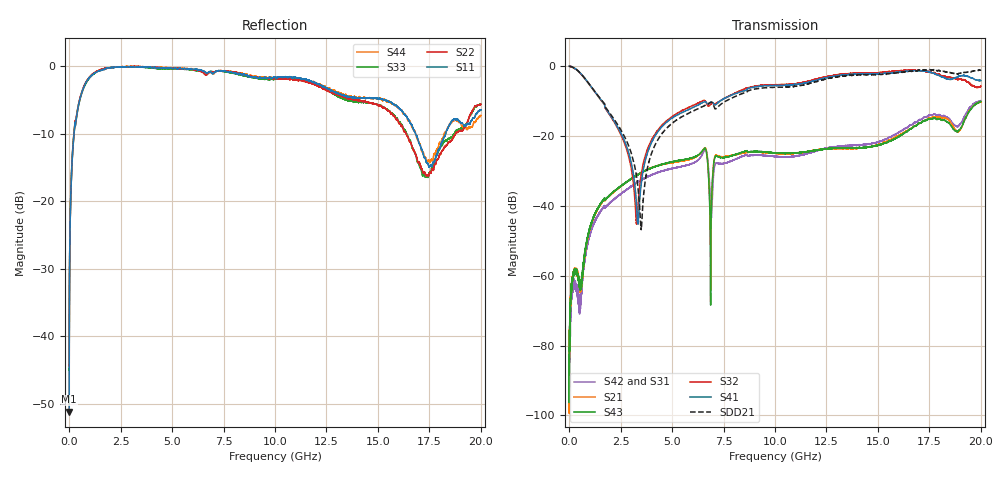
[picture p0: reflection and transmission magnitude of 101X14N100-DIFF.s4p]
!{101X14N100}
!Johanson Technology Inc.
!www.johansontechnology.com
!Test Board Conditions:
!Substrate Type  RO4350B
!Substrate Thickness  10 mil
!Substrate Dk  3.66
!TL Type: GCPW
!TL Trace Width  20 mil
!TL Gap  15 mil
!PART MODE DIFFERENTIAL
!DUT TOPOLOGY	DIFFERENTIAL 4-PORT
!Mounting Pad LxW  20x35 mil
# MHz S  dB  R 50
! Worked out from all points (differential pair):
!   20001 points, 300 kHz to 20 GHz, reference 50 ohm
!   strongest paths, dB at 300 kHz, 5 GHz, 10 GHz, 15 GHz, 20 GHz:
!     S41: 0.0, -14.9, -5.5, -2.2, -4.1
!     S32: 0.0, -14.5, -5.3, -1.9, -5.7
!     S43: -87.1, -27.4, -24.8, -22.7, -10.1
!     S21: -85.9, -27.6, -24.9, -22.6, -10.3
!     S42: -80.8, -29.3, -25.8, -21.8, -9.9
!     S31: -74.6, -29.4, -25.7, -21.8, -10.1
!   taken as a pair (ports 1,2 in; 4,3 out), SDD21 dB: 0.0, -16.4, -6.0, -2.4, -1.1
!   lowest |S11| = -51.1 dB at 1.3 MHz (marker M1), VSWR 1.01, Z = 50.1 - j0.254 ohm
!   |S11| at or under -10 dB: start of sweep to 237.8 MHz; 16.83 GHz to 18.29 GHz (1.46 GHz wide, 8.32 % of centre); 18.28786 GHz to 18.28805 GHz (187.9 kHz wide, 0.00103 % of centre)
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0.3  -51.00 -16.2  -85.28 164.2  -79.63 16.6  -0.00 -0.2
     -85.92 -132.7  -44.18 2.4  -0.01 -0.2  -87.12 -155.3
     -74.56 -13.4  -0.03 -0.3  -44.80 -2.9  -80.59 -88.7
     0.00 -0.1  -80.80 68.5  -87.15 159.6  -51.02 -17.7
1.3  -51.14 -66.0  -87.85 125.6  -86.01 -99.6  -0.01 -0.2
     -99.38 -95.9  -44.41 -22.0  -0.06 -0.0  -84.72 -100.0
     -87.78 115.0  -0.05 -0.1  -45.09 -22.9  -81.50 -7.1
     -0.01 -0.2  -87.43 -83.0  -84.25 -17.6  -51.38 -65.2
553.292  -4.49 -131.2  -64.54 81.3  -67.35 -105.6  -1.99 -41.7
         -64.19 74.3  -4.41 -133.0  -2.12 -42.6  -67.09 -102.9
         -66.08 -93.6  -2.11 -42.7  -4.60 -133.0  -62.52 85.2
         -2.00 -41.8  -66.23 -91.1  -62.55 89.7  -4.46 -133.3
3343.25  -0.10 171.4  -30.99 77.8  -33.10 76.9  -44.96 -10.0
         -31.01 77.7  -0.05 168.5  -40.21 42.8  -33.20 76.8
         -33.17 77.3  -40.23 42.9  -0.08 167.5  -31.09 76.7
         -45.09 -10.6  -33.18 76.9  -31.10 76.5  -0.09 169.3
6516.202  -0.72 134.6  -23.86 10.7  -24.71 1.5  -10.32 37.1
          -23.90 10.7  -0.93 131.3  -9.87 32.4  -24.75 -0.1
          -24.71 1.6  -9.85 32.8  -0.92 127.8  -23.89 7.2
          -10.33 37.1  -24.75 0.4  -23.92 7.2  -0.79 129.6
6875.197  -0.84 136.8  -63.98 173.3  -39.23 -123.6  -10.30 32.6
          -63.07 179.9  -0.83 129.2  -10.94 29.6  -39.67 -125.2
          -39.16 -122.4  -10.96 29.7  -0.77 126.3  -62.44 65.4
          -10.28 32.9  -39.79 -124.3  -61.21 72.2  -0.91 126.5
20000  -6.44 72.7  -10.26 104.5  -10.13 105.7  -4.14 -69.5
       -10.26 104.4  -5.65 78.8  -5.70 -71.6  -9.89 102.2
       -10.11 106.3  -5.68 -71.0  -5.62 68.8  -10.08 96.8
       -4.13 -69.2  -9.89 102.5  -10.11 96.4  -7.28 58.1
